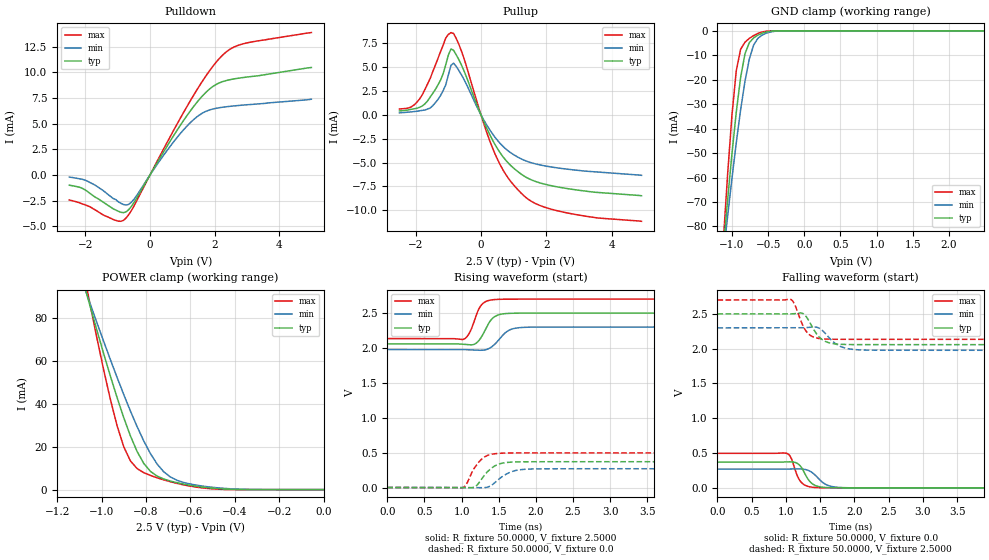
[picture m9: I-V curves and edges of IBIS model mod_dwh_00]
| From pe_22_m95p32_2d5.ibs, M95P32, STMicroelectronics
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|   Model mod_dwh_00
[Model]   mod_dwh_00
Model_type I/O
Polarity   Non-Inverting
Enable   Active-High
Vinl   =   0.750V
Vinh   =   1.750V
Vmeas  =   1.250V
Cref   =   30.0pF
C_comp   1.219pF   1.164pF   1.337pF
[Model Spec]
Vinl   0.750V  0.690V  0.810V  | <- for Vcc = 2.5V, 2.3V, 2.7V
Vinh   1.750V  1.610V  1.890V  | <- for Vcc = 2.5V, 2.3V, 2.7V
Vmeas  1.250V  1.150V  1.350V  | <- for Vcc = 2.5V, 2.3V, 2.7V
[Temperature Range]  25.0000   0.1050k   -40.0000
[Voltage Range]   2.5000V   2.3000V   2.7000V
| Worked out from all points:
|   slope of the pulldown table from 0 to 0.375 V, typ, clamps not added: 187 ohm
|   slope of the pullup table from 0 to 0.375 V, typ, clamps not added: 136 ohm
|   GND clamp passes 1 mA (typ) near -0.58 V on its own axis
|   POWER clamp passes 1 mA (typ) near -0.53 V on its own axis
|   rising waveform, R_fixture 50.0000, V_fixture 2.5000: 20-80 % time 144ps typ, 175ps min, 126ps max; typ from 2.06 V to 2.5 V
|   rising waveform, R_fixture 50.0000, V_fixture 0.0: 20-80 % time 188ps typ, 215ps min, 171ps max; typ from 0 V to 0.37 V
|   falling waveform, R_fixture 50.0000, V_fixture 0.0: 20-80 % time 142ps typ, 185ps min, 119ps max; typ from 0.37 V to 0 V
|   falling waveform, R_fixture 50.0000, V_fixture 2.5000: 20-80 % time 181ps typ, 216ps min, 149ps max; typ from 2.5 V to 2.06 V
[Pulldown]
|Voltage   I(typ)   I(min)   I(max)
-2.5V     -1mA       -211uA     -2.44mA
-1.94V    -1.6mA     -600uA     -3mA
-1.14V    -3.3mA     -2.3mA     -4.34mA
-820mV    -3.671mA   -2.881mA   -4.422mA
-660mV    -3.381mA   -2.866mA   -3.874mA
-500mV    -2.717mA   -2.383mA   -3.049mA
540mV     2.86mA     2.432mA    3.23mA
1.26V     6.286mA    5.126mA    7.287mA
1.74V     8.074mA    6.21mA     9.684mA
2.22V     9.063mA    6.585mA    11.59mA
2.86V     9.485mA    6.802mA    12.76mA
5V        10.47mA    7.38mA     13.88mA
[Pullup]
|Voltage   I(typ)   I(min)   I(max)
-2.5V     426uA      220uA      626uA
-1.96V    703uA      390uA      1.354mA
-1.48V    2.26mA     966uA      4.514mA
-1.08V    5.277mA    3.166mA    8.065mA
-920mV    6.92mA     5.2mA      8.64mA
-840mV    6.777mA    5.43mA     8.541mA
-600mV    5.245mA    4.21mA     6.715mA
440mV     -3.164mA   -2.384mA   -4.16mA
760mV     -4.751mA   -3.563mA   -6.244mA
1.24V     -6.223mA   -4.616mA   -8.228mA
2.36V     -7.554mA   -5.558mA   -10.06mA
4.92V     -8.47mA    -6.33mA    -11.15mA
[GND_clamp]
|Voltage   I(typ)   I(min)   I(max)
-2.5V     -618.8mA   -507.1mA   -839.7mA
-1.12V    -89.51mA   -92.19mA   -86.51mA
-1.06V    -69.34mA   -76.02mA   -58.94mA
-1V       -50.38mA   -60.48mA   -34.64mA
-940mV    -33.28mA   -45.81mA   -16.38mA
-880mV    -19.11mA   -32.38mA   -7.564mA
-820mV    -9.453mA   -20.71mA   -4.67mA
-760mV    -4.854mA   -11.6mA    -3.093mA
-700mV    -2.891mA   -5.814mA   -1.933mA
-580mV    -964.2uA   -1.685mA   -447.5uA
-340mV    -4.19uA    -39.9uA    -134.6nA
2.48V     343.3pA    931.5nA    131.5pA
[POWER_clamp]
|Voltage   I(typ)   I(min)   I(max)
-2.49V    667.2mA    541mA      921mA
-1.08V    96.07mA    95.11mA    101.2mA
-1.05V    84.91mA    86.28mA    85.45mA
-990mV    63.23mA    68.98mA    55.57mA
-930mV    42.88mA    52.31mA    29.76mA
-900mV    33.53mA    44.31mA    19.96mA
-840mV    17.8mA     29.4mA     9.816mA
-810mV    12.22mA    22.72mA    7.905mA
-750mV    6.305mA    11.96mA    5.516mA
-660mV    3.226mA    4.34mA     2.89mA
-420mV    154.8uA    392.4uA    29.01uA
0V        492.2pA    14.11nA    240.5pA
[Ramp]
| variable   typ   min   max
dV/dt_r   0.2219/0.2360n   0.1670/0.3005n   0.2979/0.2256n
dV/dt_f   0.2651/0.2780n   0.2003/0.3260n   0.3391/0.2713n
R_load = 50.0000
[Rising Waveform]
R_fixture= 50.0000
V_fixture= 2.5000
V_fixture_min= 2.3000
V_fixture_max= 2.7000
|time   V(typ)   V(min)   V(max)
0s        2.058V     1.978V     2.135V
1.024ns   2.053V     1.977V     2.124V
1.104ns   2.046V     1.974V     2.213V
1.184ns   2.061V     1.969V     2.429V
1.256ns   2.14V      1.967V     2.602V
1.376ns   2.373V     1.997V     2.684V
1.456ns   2.456V     2.064V     2.695V
1.632ns   2.496V     2.251V     2.7V
1.872ns   2.5V       2.297V     2.7V
8ns       2.5V       2.3V       2.7V
[Rising Waveform]
R_fixture= 50.0000
V_fixture= 0.0
V_fixture_min= 0.0
V_fixture_max= 0.0
|time   V(typ)   V(min)   V(max)
0s        8.608nV    979.2nV    1.51nV
1.024ns   -565.9uV   253.8uV    1.551mV
1.072ns   -1.939mV   182.5uV    62.4mV
1.168ns   4.755mV    -713.2uV   273.1mV
1.264ns   114.8mV    -3.095mV   401.9mV
1.376ns   254.4mV    16.73mV    469.7mV
1.52ns    342mV      136.1mV    491.2mV
1.712ns   366.2mV    240.1mV    495.8mV
1.984ns   369.6mV    267mV      496.4mV
8ns       369.9mV    269.2mV    496.4mV
[Falling Waveform]
R_fixture= 50.0000
V_fixture= 0.0
V_fixture_min= 0.0
V_fixture_max= 0.0
|time   V(typ)   V(min)   V(max)
0s        369.9mV    269.2mV    496.4mV
1.016ns   373.3mV    269.9mV    494.2mV
1.08ns    373.8mV    271.2mV    419.6mV
1.168ns   350.6mV    272.8mV    169.5mV
1.224ns   295.8mV    271.3mV    79.33mV
1.336ns   106.5mV    246.4mV    17.45mV
1.432ns   33.05mV    178.4mV    4.806mV
1.608ns   3.826mV    37.23mV    471.9uV
1.864ns   185.2uV    2.507mV    20.23uV
8ns       465.7nV    1.371uV    556.4nV
[Falling Waveform]
R_fixture= 50.0000
V_fixture= 2.5000
V_fixture_min= 2.3000
V_fixture_max= 2.7000
|time   V(typ)   V(min)   V(max)
0s        2.5V       2.3V       2.7V
1.08ns    2.501V     2.3V       2.704V
1.128ns   2.504V     2.3V       2.634V
1.24ns    2.509V     2.302V     2.347V
1.304ns   2.45V      2.304V     2.239V
1.448ns   2.212V     2.309V     2.154V
1.544ns   2.122V     2.251V     2.141V
1.784ns   2.064V     2.038V     2.135V
2.088ns   2.059V     1.983V     2.135V
8ns       2.058V     1.978V     2.135V
